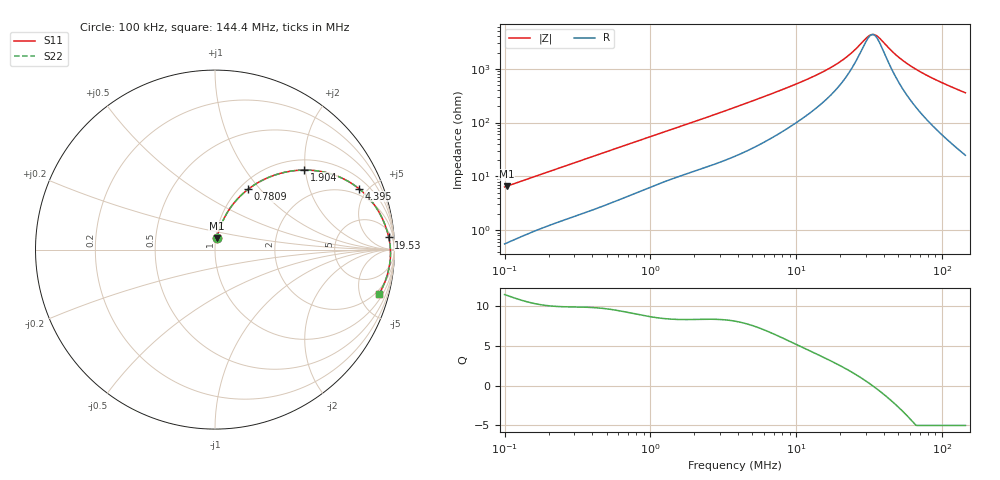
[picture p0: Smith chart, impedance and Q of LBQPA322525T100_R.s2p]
! LBQPA322525T100_R  S-PARAMETER MODEL  ( General Type )
! Model Generated by TAIYO YUDEN Corporation (http://www.ty-top.com)
! Version 1.0
! TAIYO YUDEN Control No. 191025NI43SB-FBB
! Copyright(c) 2019 TAIYO YUDEN CO.,LTD. All Rights Reserved.
! Product Description (link to TY-COMPAS)
! https://ds.yuden.co.jp/TYCOMPAS/or/detail?pn=LBQPA322525T100KR&u=M
! Products Name : Inductors
! Characteristics :
!  Inductance : 10 uH , SRF(min) : 23 MHz , DC Resistance(max) : 0.1729 Ohm
!  Rated Current : Saturation :900 mA , Temp Rise : 720 mA (20 degC)
!  Case Size : 3.2 x 2.5 / 0.126 x 0.098 [mm/inch] , Thickness : 2.5 / 0.098 [mm/inch]
!  (Conditions: Temperature = 25 degC , DC Bias Current/Voltage = 0A / 0V)
! External Node Assignments :
!  1  o---GGG---o  2
! GND o---------o GND
! Frequency Range : 0.1MHz  -  144.390904MHz  [ 402 STEP ]
# MHz S RI R 50
! Freq[MHz].  S11 Real  S11 Imag  S21 Real  S21 Imag  S12 Real  S12 Imag  S22 Real  S22 Imag
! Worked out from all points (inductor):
!   401 points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, 100 kHz to 144.4 MHz, reference 50 ohm
!   read as one part in series: L = 9.92 uH near 103.7 kHz
!   highest Q = 11.3 at 103.7 kHz (marker M1), where L = 10 uH
!   self-resonance near 33.24 MHz
!   S11 on the Smith chart (normalised r, x): 100 kHz: 1.01, +0.13; 780.9 kHz: 1.10, +0.87; 1.904 MHz: 1.24, +1.97; 4.395 MHz: 1.56, +4.40; 19.53 MHz: 10, +24; 144.4 MHz: 1.49, -7.14
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0.1  0.00944 0.0623  0.9906 -0.0623  0.9906 -0.0623  0.00944 0.0623
0.103705  0.00996 0.0645  0.99 -0.0645  0.99 -0.0645  0.00996 0.0645
0.338238  0.0552 0.183  0.9448 -0.183  0.9448 -0.183  0.0552 0.183
0.780854  0.1852 0.3367  0.8148 -0.3367  0.8148 -0.3367  0.1852 0.3367
1.144052  0.2992 0.4026  0.7008 -0.4026  0.7008 -0.4026  0.2992 0.4026
1.903766  0.497 0.4432  0.503 -0.4432  0.503 -0.4432  0.497 0.4432
2.641149  0.6313 0.426  0.3687 -0.426  0.3687 -0.426  0.6313 0.426
3.869624  0.766 0.3657  0.234 -0.3657  0.234 -0.3657  0.766 0.3657
4.395019  0.8022 0.3395  0.1978 -0.3395  0.1978 -0.3395  0.8022 0.3395
7.0523  0.8961 0.2371  0.1039 -0.2371  0.1039 -0.2371  0.8961 0.2371
12.85266  0.9509 0.1277  0.0491 -0.1277  0.0491 -0.1277  0.9509 0.1277
19.52839  0.9682 0.0678  0.0318 -0.0678  0.0318 -0.0678  0.9682 0.0678
23.42367  0.9727 0.0442  0.0273 -0.0442  0.0273 -0.0442  0.9727 0.0442
30.21613  0.9767 0.012  0.0233 -0.012  0.0233 -0.012  0.9767 0.012
32.49632  0.9773 0.00284  0.0227 -0.00284  0.0227 -0.00284  0.9773 0.00284
34.31869  0.9776 -0.00407  0.0224 0.00407  0.0224 0.00407  0.9776 -0.00407
36.24326  0.9779 -0.011  0.0221 0.011  0.0221 0.011  0.9779 -0.011
43.47261  0.9777 -0.0348  0.0223 0.0348  0.0223 0.0348  0.9777 -0.0348
54.07568  0.9754 -0.065  0.0246 0.065  0.0246 0.065  0.9754 -0.065
69.75669  0.9692 -0.104  0.0308 0.104  0.0308 0.104  0.9692 -0.104
98.55167  0.9519 -0.166  0.0481 0.166  0.0481 0.166  0.9519 -0.166
144.3909  0.9128 -0.2497  0.0872 0.2497  0.0872 0.2497  0.9128 -0.2497
